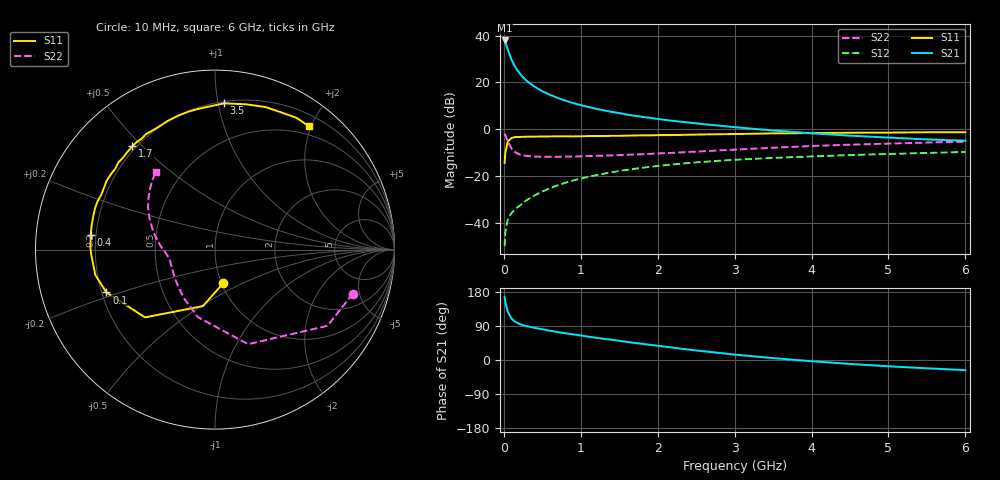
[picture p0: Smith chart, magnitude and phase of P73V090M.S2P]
! SIEMENS Small Signal Semiconductors
! BFP196
! Si NPN RF Bipolar Junction Transistor in SOT143
! VCE = 3 V  IC = 90 mA
! Common Emitter S-Parameters:  May  1996
# GHz  S  MA  R  50
!  f  S11  S21  S12  S22
! GHz  MAG  ANG  MAG  ANG  MAG  ANG  MAG  ANG
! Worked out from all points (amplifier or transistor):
!   36 points, 10 MHz to 6 GHz, reference 50 ohm
!   highest |S21| = 37.9 dB at 10 MHz (marker M1)
!   |S21| within 3 dB of that: start of sweep to 42.44 MHz
!   unconditionally stable (mu >= 1): 329.3 MHz to 4.443 GHz
!   at 250 MHz: K = 0.95, MSG = 26.8 dB, |S12| = -31.4 dB
!   at 1.4 GHz: K = 1.09, MAG = 11.1 dB, |S12| = -18.4 dB
!   at 6 GHz: K = 0.98, MSG = 2.4 dB, |S12| = -9.7 dB
!   S11 on the Smith chart (normalised r, x): 10 MHz: 1.02, -0.39; 100 MHz: 0.22, -0.18; 400 MHz: 0.18, +0.06; 1.7 GHz: 0.19, +0.47; 3.5 GHz: 0.21, +1.04; 6 GHz: 0.36, +1.96
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0.01  0.1912 -75.7  78.56 166.1  0.0032 75.5  0.8064 -17.7
0.02  0.3218 -102.0  72.17 152.8  0.0065 67.5  0.757 -34.1
0.05  0.5427 -135.9  50.94 127.7  0.0117 51.9  0.5585 -70.7
0.1  0.6505 -158.5  30.26 109.2  0.0164 51.3  0.3884 -104.1
0.15  0.6814 -168.0  21.01 100.7  0.02 55.2  0.3223 -122.3
0.2  0.6849 -174.1  16.03 95.4  0.023 58.1  0.2929 -133.7
0.25  0.6906 -178.0  12.82 91.8  0.0268 60.8  0.2778 -142.0
0.3  0.6943 179.0  10.73 89.2  0.031 62.4  0.2702 -147.4
0.4  0.6974 173.2  8.116 84.8  0.0388 65.1  0.2619 -155.3
0.5  0.7002 169.3  6.486 81.0  0.0467 66.2  0.2589 -160.3
0.6  0.7032 165.1  5.421 77.3  0.0555 66.4  0.2584 -163.6
0.7  0.7066 161.1  4.657 73.6  0.0637 66.1  0.2589 -166.2
0.9  0.7035 154.3  3.626 67.6  0.0808 64.3  0.2618 -170.2
1.1  0.7157 147.6  2.981 61.6  0.0969 62.1  0.2679 -173.0
1.3  0.7159 140.9  2.531 55.9  0.1128 59.3  0.2737 -175.7
1.7  0.7371 128.7  1.944 45.1  0.1435 53.7  0.2895 179.4
2.2  0.7512 115.4  1.51 32.7  0.1778 45.8  0.3145 173.4
3  0.7905 96.1  1.108 14.2  0.2233 33.5  0.367 161.7
3.5  0.8169 86.4  0.941 5.0  0.245 26.4  0.4034 154.6
4.5  0.8426 70.4  0.731 -10.4  0.2816 14.2  0.4688 142.3
5.5  0.8631 58.3  0.607 -21.9  0.3126 3.4  0.5208 132.1
6  0.8636 52.9  0.57 -26.8  0.3276 -2.3  0.5457 127.2
